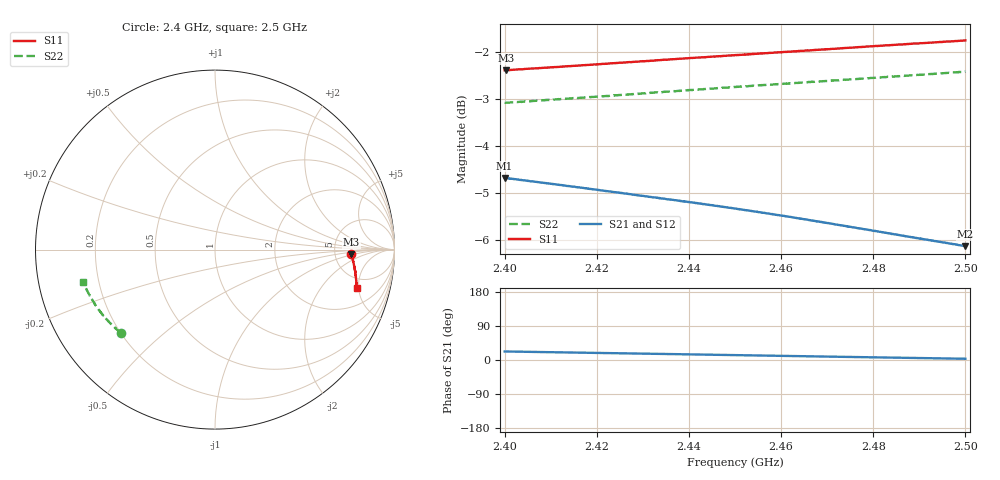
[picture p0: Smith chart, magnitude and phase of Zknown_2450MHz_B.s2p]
!Agilent Technologies,N5242A,MY49421279,A.09.90.21
!Agilent N5242A: A.09.90.21
!Date: Monday, January 30, 2023
!Caliblation kit: 85033D 3.5mm Calibration Kit
!DUT Connector Gender Port1: male
!DUT Connector Gender Port2: female
!S2P File: Measurements: S11, S21, S12, S22:
# Hz S  dB  R 50
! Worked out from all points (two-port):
!   1001 points, 2.4 GHz to 2.5 GHz, reference 50 ohm
!   highest |S21| = -4.68 dB at 2.4 GHz (marker M1); lowest = -6.1 dB at 2.4999 GHz (marker M2)
!   |S21| within 3 dB of the highest: start of sweep to end of sweep
!   lowest |S11| = -2.4 dB at 2.4003 GHz (marker M3), VSWR 7.31, Z = 360 - j44.4 ohm
!   |S11| at or under -10 dB: nowhere
!   |S22| runs from -3.1 to -2.4 dB; largest |S21 - S12| = 0.004
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2.4e9  -2.39 -2.0  -4.68 22.5  -4.65 22.3  -3.09 -138.7
2.4003e9  -2.39 -2.0  -4.69 22.5  -4.65 22.2  -3.08 -138.7
2.4058e9  -2.36 -2.7  -4.76 21.4  -4.72 21.2  -3.05 -140.2
2.4075e9  -2.34 -2.9  -4.78 21.1  -4.74 20.9  -3.04 -140.7
2.4126e9  -2.31 -3.5  -4.84 20.1  -4.80 19.9  -3.00 -142.1
2.4167e9  -2.29 -4.0  -4.89 19.4  -4.86 19.1  -2.98 -143.3
2.4253e9  -2.23 -5.1  -5.00 17.7  -4.96 17.5  -2.92 -145.6
2.4314e9  -2.19 -5.9  -5.09 16.5  -5.05 16.3  -2.88 -147.3
2.4334e9  -2.18 -6.2  -5.12 16.1  -5.08 15.9  -2.86 -147.8
2.4354e9  -2.16 -6.4  -5.14 15.8  -5.10 15.5  -2.85 -148.4
2.44e9  -2.13 -7.0  -5.20 14.9  -5.16 14.6  -2.81 -149.7
2.45e9  -2.07 -8.3  -5.34 12.9  -5.31 12.7  -2.75 -152.4
2.4568e9  -2.03 -9.2  -5.44 11.6  -5.40 11.3  -2.70 -154.4
2.4609e9  -2.00 -9.7  -5.50 10.7  -5.47 10.5  -2.68 -155.5
2.4667e9  -1.97 -10.5  -5.60 9.6  -5.56 9.4  -2.63 -157.1
2.4733e9  -1.92 -11.4  -5.70 8.4  -5.66 8.1  -2.60 -158.9
2.4834e9  -1.86 -12.7  -5.87 6.4  -5.83 6.1  -2.53 -161.7
2.4921e9  -1.80 -14.0  -6.01 4.8  -5.98 4.5  -2.47 -164.1
2.498e9  -1.77 -14.7  -6.11 3.6  -6.08 3.3  -2.43 -165.7
2.4993e9  -1.76 -14.9  -6.13 3.4  -6.10 3.0  -2.42 -166.1
2.4999e9  -1.76 -15.0  -6.14 3.2  -6.11 2.9  -2.42 -166.2
2.5e9  -1.76 -15.0  -6.14 3.2  -6.12 2.9  -2.42 -166.3
